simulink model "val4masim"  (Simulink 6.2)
settings: Solver=ode4  SolverMode=SingleTasking  StartTime=0  StopTime=150  FixedStep=0.0025  RelTol=1e-3  AbsTol=1e-6
libraries: DABLib x3, simulink x1

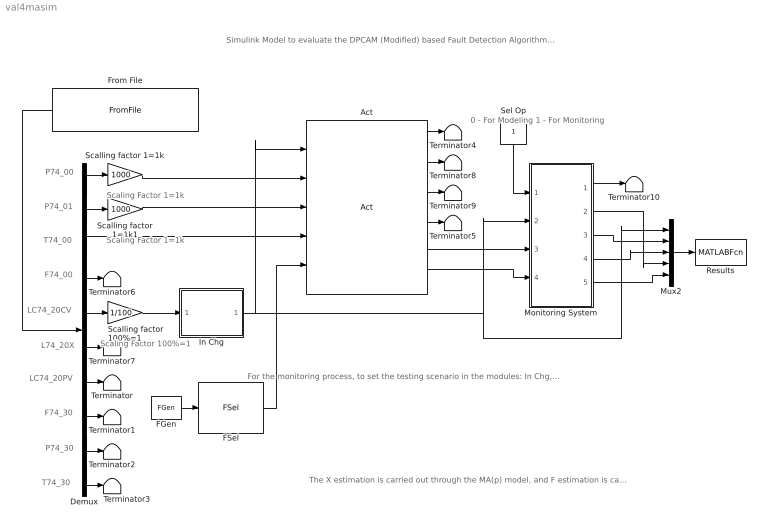
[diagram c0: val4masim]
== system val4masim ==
  note: P74_00
  note: P74_01
  note: T74_00
  note: F74_00
  note: LC74_20CV
  note: L74_20X
  note: LC74_20PV
  note: F74_30
  note: P74_30
  note: T74_30
  note: For the monitoring process, to set the testing scenario in the modules: In Chg, FGen, FSel
  note: Scaling Factor 1=1k
  note: Scaling Factor 1=1k
  note: Scaling Factor 100%=1
  note: Simulink Model to evaluate the DPCAM (Modified) based Fault Detection Algorithm This model is controlled from the User Interface - Val4 Mon.fig
  note: The X estimation is carried out through the MA(p) model, and F estimation is carried out through the flow characteristic empirical model The auto-correlation and cross-correlation coefficients, from Correlation Matrix used in the Statistical Model, are used to obtain the parameters phi of MA(p) model
  note: 0 - For Modeling 1 - For Monitoring
  Act : DABLib/Act  Dist=on
  Demux : Demux  Outputs=10
  FGen : DABLib/FGen  From=100  To=inf  MFS=0.5  FDT=0  FSD=1
  FSel : DABLib/FSel  FSel=f3 - Valve plug or valve seat erosion
  From File : FromFile  Orientation=left  FileName=OneHourTestData_ExampleII.mat
  In Chg : Subsystem
  Monitoring System : Subsystem
  Mux2 : Mux  Inputs=5
  Results : MATLABFcn  MATLABFcn=Resongui_Val4  OutputDimensions=0  OutputSignalType=real  Output1D=off  SampleTime=0.1
  Scalling factor 100%=1 : Gain  Gain=1/100
  Scalling factor 1=1k : Gain  Gain=1000
  Scalling factor 1=1k1 : Gain  Gain=1000
  Sel Op : Constant  Orientation=down
  Terminator{,1..10} (11 alike) : Terminator
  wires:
  FGen/1 -> FSel/1
  FSel/1 -> Act/5
  Act/4 -> Terminator5/1
  Act/1 -> Terminator4/1
  From File/1 -> Demux/1
  Demux/9 -> Terminator2/1
  Demux/8 -> Terminator1/1
  Demux/7 -> Terminator/1
  Demux/5 -> Scalling factor 100%=1/1
  Demux/1 -> Scalling factor 1=1k/1
  Demux/2 -> Scalling factor 1=1k1/1
  Scalling factor 1=1k/1 -> Act/2
  Scalling factor 1=1k1/1 -> Act/3
  Demux/3 -> Act/4
  Demux/6 -> Terminator7/1
  Demux/10 -> Terminator3/1
  Scalling factor 100%=1/1 -> In Chg/1(CV)
  Demux/4 -> Terminator6/1
  Act/2 -> Terminator8/1
  Act/3 -> Terminator9/1
  Act/5 -> Monitoring System/3(X)
  Act/6 -> Monitoring System/4(F)
  In Chg/1(CV+Per) -> Act/1, Monitoring System/2(CV), Mux2/1
  Sel Op/1 -> Monitoring System/1(Sel)
  Monitoring System/4(F / Fest) -> Mux2/3
  Monitoring System/3(X / Xest) -> Mux2/2
  Monitoring System/2(Mon2) -> Mux2/4
  Mux2/1 -> Results/1
  Monitoring System/5(Time) -> Mux2/5
  Monitoring System/1(Mon1) -> Terminator10/1

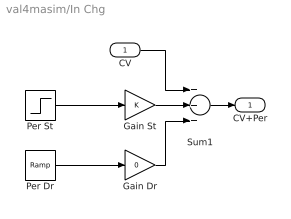
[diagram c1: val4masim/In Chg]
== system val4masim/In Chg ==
  CV : Inport  Port=1  LatchInput=off
  Gain Dr : Gain  Gain=0
  Gain St : Gain
  Per Dr : simulink/Sources/Ramp  slope=0.002  start=70  X0=0
  Per St : Step  Time=70  After=0.1
  Sum1 : Sum  Inputs=+++
  CV+Per : Outport
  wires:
  CV/1 -> Sum1/1
  Sum1/1 -> CV+Per/1
  Gain St/1 -> Sum1/2
  Gain Dr/1 -> Sum1/3
  Per St/1 -> Gain St/1
  Per Dr/1 -> Gain Dr/1

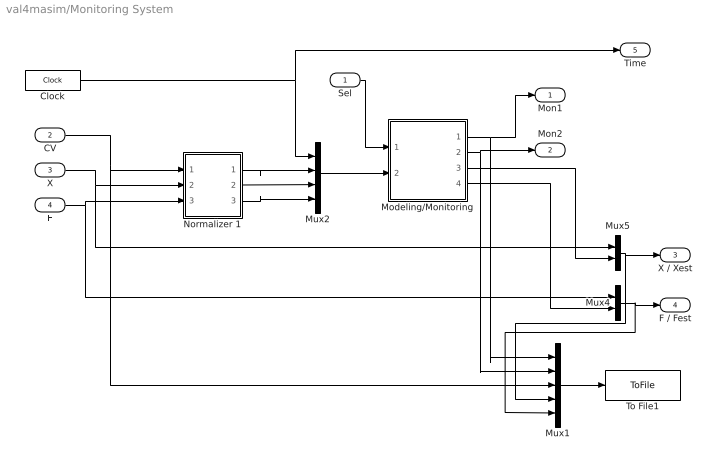
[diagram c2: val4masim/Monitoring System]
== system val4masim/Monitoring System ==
  Sel : Inport  Port=1  LatchInput=off
  CV : Inport  Port=2  LatchInput=off
  X : Inport  Port=3  LatchInput=off
  F : Inport  Port=4  LatchInput=off
  Clock : Clock
  Modeling/Monitoring : Subsystem
  Mux1 : Mux  Inputs=5
  Mux2 : Mux
  Mux4 : Mux  Inputs=2
  Mux5 : Mux  Inputs=2
  Normalizer 1 : Subsystem
  To File1 : ToFile  Filename=DataPlot  MatrixName=DP  SampleTime=0.5
  Mon1 : Outport
  Mon2 : Outport  Port=2
  X / Xest : Outport  Port=3
  F / Fest : Outport  Port=4
  Time : Outport  Port=5
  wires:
  F/1 -> Mux4/1, Normalizer 1/3(Q)
  Clock/1 -> Mux2/1, Time/1
  Mux2/1 -> Modeling/Monitoring/2(Data)
  Modeling/Monitoring/1(Mon1) -> Mon1/1, Mux1/1
  Modeling/Monitoring/2(Mon2) -> Mon2/1, Mux1/2
  Mux5/1 -> Mux1/4, X / Xest/1
  Mux4/1 -> F / Fest/1, Mux1/5
  Sel/1 -> Modeling/Monitoring/1(Sel)
  X/1 -> Mux5/1, Normalizer 1/2(X)
  Mux1/1 -> To File1/1
  CV/1 -> Mux1/3, Normalizer 1/1(CV)
  Modeling/Monitoring/3(Xest) -> Mux5/2
  Modeling/Monitoring/4(Fest) -> Mux4/2
  Normalizer 1/3(Qt) -> Mux2/4
  Normalizer 1/2(Xt) -> Mux2/3
  Normalizer 1/1(CVt) -> Mux2/2

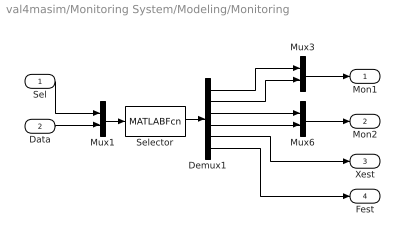
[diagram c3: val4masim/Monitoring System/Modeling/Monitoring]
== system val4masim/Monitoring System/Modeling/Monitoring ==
  Sel : Inport  Port=1  LatchInput=off
  Data : Inport  Port=2  LatchInput=off
  Demux1 : Demux  Outputs=6
  Mux1 : Mux  Inputs=2
  Mux3 : Mux  Inputs=2
  Mux6 : Mux  Inputs=2
  Selector : MATLABFcn  MATLABFcn=FunSel_Val4  OutputDimensions=6  OutputSignalType=real  Output1D=off  SampleTime=0.5
  Mon1 : Outport
  Mon2 : Outport  Port=2
  Xest : Outport  Port=3
  Fest : Outport  Port=4
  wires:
  Mux1/1 -> Selector/1
  Selector/1 -> Demux1/1
  Mux3/1 -> Mon1/1
  Sel/1 -> Mux1/1
  Mux6/1 -> Mon2/1
  Data/1 -> Mux1/2
  Demux1/1 -> Mux3/1
  Demux1/2 -> Mux3/2
  Demux1/3 -> Mux6/1
  Demux1/4 -> Mux6/2
  Demux1/5 -> Xest/1
  Demux1/6 -> Fest/1

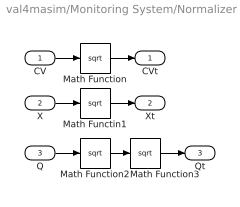
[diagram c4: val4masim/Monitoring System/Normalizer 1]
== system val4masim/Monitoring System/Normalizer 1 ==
  CV : Inport  Port=1  LatchInput=off
  X : Inport  Port=2  LatchInput=off
  Q : Inport  Port=3  LatchInput=off
  Math Functin1 : Math  Operator=sqrt
  Math Function : Math  Operator=sqrt
  Math Function2 : Math  Operator=sqrt
  Math Function3 : Math  Operator=sqrt
  CVt : Outport
  Xt : Outport  Port=2
  Qt : Outport  Port=3
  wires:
  Math Function2/1 -> Math Function3/1
  CV/1 -> Math Function/1
  Math Function/1 -> CVt/1
  X/1 -> Math Functin1/1
  Math Functin1/1 -> Xt/1
  Q/1 -> Math Function2/1
  Math Function3/1 -> Qt/1
